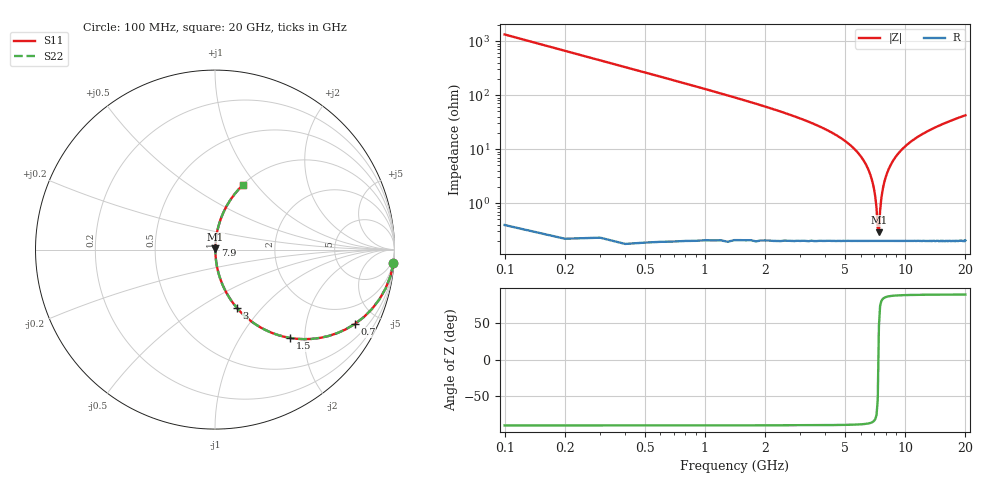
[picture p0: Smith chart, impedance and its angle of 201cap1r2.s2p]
! AVX Thin Film Operation		Date: May 2007
! Description: Accu-P® Series, Thin Film, SMD, RF Capacitor
! Part Number: 02013J1R2ABS
! 50 MHz  -  20.05 GHz
! Serial Measurements
# hz S db R 50
!	S11		S21		S12		S22
!	dB	Phase	dB	Phase	dB	Phase	dB	Phase
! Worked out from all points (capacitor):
!   200 points, 100 MHz to 20 GHz, reference 50 ohm
!   read as one part in series: C = 1.2 pF near 200 MHz
!   lowest |Z| = 290 mohm at 7.4 GHz (marker M1)
!   series resonance near 7.357 GHz, so ESL is about 390 pH
!   S11 on the Smith chart (normalised r, x): 100 MHz: 1, -27; 700 MHz: 1.00, -3.75; 1.5 GHz: 1.00, -1.69; 3 GHz: 1.00, -0.74; 7.9 GHz: 1.00, +0.05; 20 GHz: 1.00, +0.85
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1e8  -0.02 -4.3  -22.48 85.7  -22.48 85.7  -0.02 -4.3
2e8  -0.10 -8.6  -16.52 81.4  -16.52 81.4  -0.10 -8.6
3e8  -0.22 -12.8  -13.11 77.2  -13.11 77.2  -0.22 -12.8
7e8  -1.09 -28.0  -6.56 61.9  -6.56 61.9  -1.09 -28.0
1.5e9  -3.80 -49.6  -2.36 40.2  -2.36 40.2  -3.80 -49.6
3e9  -9.24 -69.5  -0.57 20.2  -0.57 20.2  -9.24 -69.5
3.5e9  -11.03 -73.3  -0.37 16.3  -0.37 16.3  -11.03 -73.3
5.7e9  -20.68 -83.5  -0.05 5.3  -0.05 5.3  -20.68 -83.5
6.4e9  -25.97 -84.8  -0.03 2.9  -0.03 2.9  -25.97 -84.8
6.8e9  -30.93 -84.3  -0.02 1.6  -0.02 1.6  -30.93 -84.3
7.1e9  -37.76 -80.4  -0.02 0.7  -0.02 0.7  -37.76 -80.4
7.2e9  -41.92 -75.1  -0.02 0.4  -0.02 0.4  -41.92 -75.1
7.3e9  -49.28 -54.3  -0.02 0.2  -0.02 0.2  -49.28 -54.3
7.4e9  -50.76 46.3  -0.02 -0.1  -0.02 -0.1  -50.76 46.3
7.5e9  -42.84 73.5  -0.02 -0.4  -0.02 -0.4  -42.84 73.5
7.6e9  -38.51 79.6  -0.02 -0.7  -0.02 -0.7  -38.51 79.6
7.9e9  -31.80 84.1  -0.02 -1.5  -0.02 -1.5  -31.80 84.1
8.7e9  -24.36 84.6  -0.03 -3.5  -0.03 -3.5  -24.36 84.6
1.01e10  -18.77 82.4  -0.08 -6.6  -0.08 -6.6  -18.77 82.4
1.34e10  -13.03 76.6  -0.24 -12.9  -0.24 -12.9  -13.03 76.6
1.67e10  -10.10 71.4  -0.46 -18.2  -0.46 -18.2  -10.10 71.4
2e10  -8.19 66.8  -0.73 -22.9  -0.73 -22.9  -8.19 66.8
